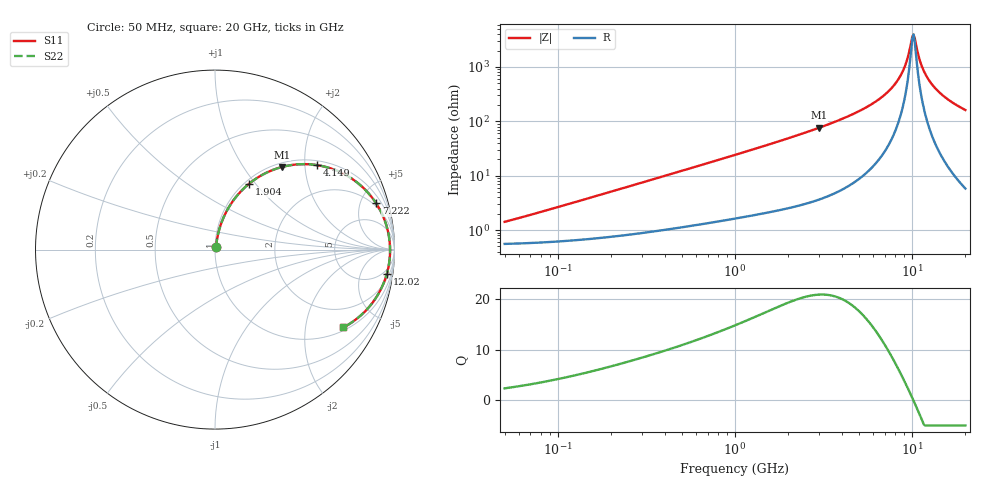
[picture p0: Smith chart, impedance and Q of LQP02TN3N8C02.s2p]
!Murata Part Number: LQP02TN3N8C02
!These Parameters are Measured in Series Mode Connection
!  o--[Z]--o
!Port1  Port2
!  o-------o
!Freq. Start=50[MHz] Stop=20[GHz], 401[Steps]
# Hz S RI R 50
!Freq.(Hz) S11(Real) S11(Imag) S21(Real) S21(Imag) S12(Real) S12(Imag) S22(Real) S22(Imag)
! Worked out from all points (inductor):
!   401 points, 50 MHz to 20 GHz, reference 50 ohm
!   read as one part in series: L = 4.11 nH near 66.46 MHz
!   highest Q = 20.9 at 2.985 GHz (marker M1), where L = 4.05 nH
!   self-resonance near 10.04 GHz
!   S11 on the Smith chart (normalised r, x): 50 MHz: 1.01, +0.03; 1.904 GHz: 1.05, +0.93; 4.149 GHz: 1.12, +2.31; 7.222 GHz: 1.66, +6.70; 12.02 GHz: 3, -14; 20 GHz: 1.12, -3.22
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5e7  0.00569 0.0129  0.9943 -0.0129  0.9943 -0.0129  0.00569 0.0129
1.364002e8  0.00779 0.0343  0.9922 -0.0343  0.9922 -0.0343  0.00779 0.0343
3.721004e8  0.0178 0.0893  0.9822 -0.0893  0.9822 -0.0893  0.0178 0.0893
1e9  0.0682 0.2206  0.9318 -0.2206  0.9318 -0.2206  0.0682 0.2206
1.904239e9  0.1891 0.3662  0.8109 -0.3662  0.8109 -0.3662  0.1891 0.3662
2.728004e9  0.3276 0.4459  0.6724 -0.4459  0.6724 -0.4459  0.3276 0.4459
2.98453e9  0.3726 0.4602  0.6274 -0.4602  0.6274 -0.4602  0.3726 0.4602
4.149438e9  0.5687 0.4706  0.4313 -0.4706  0.4313 -0.4706  0.5687 0.4706
5.683258e9  0.7715 0.389  0.2285 -0.389  0.2285 -0.389  0.7715 0.389
7.222371e9  0.8978 0.2579  0.1022 -0.2579  0.1022 -0.2579  0.8978 0.2579
7.442007e9  0.9101 0.2379  0.0899 -0.2379  0.0899 -0.2379  0.9101 0.2379
8.141811e9  0.9413 0.174  0.0587 -0.174  0.0587 -0.174  0.9413 0.174
8.774992e9  0.9599 0.1171  0.0401 -0.1171  0.0401 -0.1171  0.9599 0.1171
9.316812e9  0.9697 0.07  0.0303 -0.07  0.0303 -0.07  0.9697 0.07
9.892087e9  0.9748 0.0219  0.0252 -0.0219  0.0252 -0.0219  0.9748 0.0219
1.019291e10  0.9755 -0.00223  0.0245 0.00223  0.0245 0.00223  0.9755 -0.00223
1.050288e10  0.975 -0.0264  0.025 0.0264  0.025 0.0264  0.975 -0.0264
1.131968e10  0.9684 -0.0865  0.0316 0.0865  0.0316 0.0865  0.9684 -0.0865
1.201863e10  0.9578 -0.1337  0.0422 0.1337  0.0422 0.1337  0.9578 -0.1337
1.314879e10  0.9334 -0.2015  0.0666 0.2015  0.0666 0.2015  0.9334 -0.2015
1.482269e10  0.8863 -0.2841  0.1137 0.2841  0.1137 0.2841  0.8863 -0.2841
2e10  0.7153 -0.4336  0.2847 0.4336  0.2847 0.4336  0.7153 -0.4336
